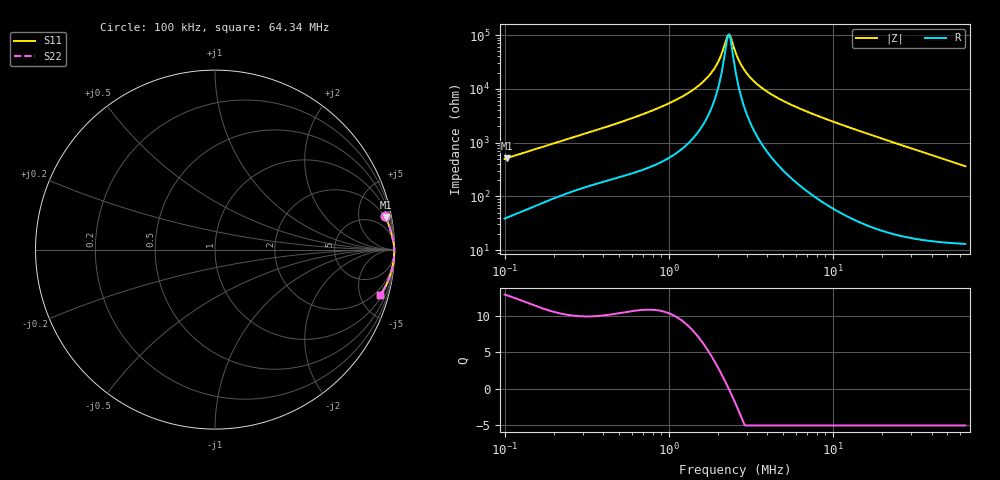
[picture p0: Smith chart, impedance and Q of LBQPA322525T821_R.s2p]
! LBQPA322525T821_R  S-PARAMETER MODEL  ( General Type )
! Model Generated by TAIYO YUDEN Corporation (http://www.ty-top.com)
! Version 1.0
! TAIYO YUDEN Control No. 191025NI43SB-FBB
! Copyright(c) 2019 TAIYO YUDEN CO.,LTD. All Rights Reserved.
! Product Description (link to TY-COMPAS)
! https://ds.yuden.co.jp/TYCOMPAS/or/detail?pn=LBQPA322525T821KR&u=M
! Products Name : Inductors
! Characteristics :
!  Inductance : 820 uH , SRF(min) : 1.8 MHz , DC Resistance(max) : 15.6 Ohm
!  Rated Current : Saturation :110 mA , Temp Rise : 80 mA (20 degC)
!  Case Size : 3.2 x 2.5 / 0.126 x 0.098 [mm/inch] , Thickness : 2.5 / 0.098 [mm/inch]
!  (Conditions: Temperature = 25 degC , DC Bias Current/Voltage = 0A / 0V)
! External Node Assignments :
!  1  o---GGG---o  2
! GND o---------o GND
! Frequency Range : 0.1MHz  -  64.339822MHz  [ 402 STEP ]
# MHz S RI R 50
! Freq[MHz].  S11 Real  S11 Imag  S21 Real  S21 Imag  S12 Real  S12 Imag  S22 Real  S22 Imag
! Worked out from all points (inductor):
!   401 points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, 100 kHz to 64.34 MHz, reference 50 ohm
!   read as one part in series: L = 782 uH near 103.3 kHz
!   highest Q = 12.8 at 103.3 kHz (marker M1), where L = 790 uH
!   self-resonance near 2.302 MHz
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0.1  0.9479 0.1867  0.0521 -0.1867  0.0521 -0.1867  0.9479 0.1867
0.103286  0.9504 0.1815  0.0496 -0.1815  0.0496 -0.1815  0.9504 0.1815
0.295407  0.988 0.0697  0.012 -0.0697  0.012 -0.0697  0.988 0.0697
0.554941  0.995 0.0376  0.00502 -0.0376  0.00502 -0.0376  0.995 0.0376
0.872651  0.9974 0.0223  0.00259 -0.0223  0.00259 -0.0223  0.9974 0.0223
1.307286  0.9985 0.012  0.00153 -0.012  0.00153 -0.012  0.9985 0.012
1.693207  0.9988 0.00638  0.00118 -0.00638  0.00118 -0.00638  0.9988 0.00638
1.86568  0.9989 0.00439  0.00109 -0.00439  0.00109 -0.00439  0.9989 0.00439
1.990316  0.999 0.00309  0.00105 -0.00309  0.00105 -0.00309  0.999 0.00309
2.089227  0.999 0.00212  0.00102 -0.00212  0.00102 -0.00212  0.999 0.00212
2.228796  0.999 0.000838  0.000985 -0.000838  0.000985 -0.000838  0.999 0.000838
2.302039  0.999 0.000197  0.000971 -0.000197  0.000971 -0.000197  0.999 0.000197
2.377689  0.999 -0.000444  0.000958 0.000444  0.000958 0.000444  0.999 -0.000444
2.53653  0.9991 -0.00173  0.000939 0.00173  0.000939 0.00173  0.9991 -0.00173
2.705981  0.9991 -0.00302  0.000926 0.00302  0.000926 0.00302  0.9991 -0.00302
2.886752  0.9991 -0.00433  0.000919 0.00433  0.000919 0.00433  0.9991 -0.00433
3.180803  0.9991 -0.00633  0.00092 0.00633  0.00092 0.00633  0.9991 -0.00633
3.561928  0.9991 -0.00873  0.000939 0.00873  0.000939 0.00873  0.9991 -0.00873
4.842704  0.9989 -0.0159  0.0011 0.0159  0.0011 0.0159  0.9989 -0.0159
7.493079  0.9983 -0.0289  0.00173 0.0289  0.00173 0.0289  0.9983 -0.0289
22.13506  0.9895 -0.0926  0.0105 0.0926  0.0105 0.0926  0.9895 -0.0926
64.33982  0.9219 -0.251  0.0781 0.251  0.0781 0.251  0.9219 -0.251
